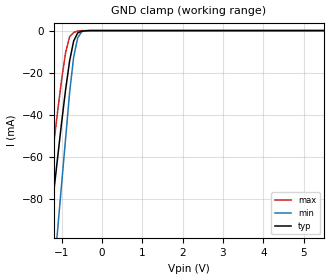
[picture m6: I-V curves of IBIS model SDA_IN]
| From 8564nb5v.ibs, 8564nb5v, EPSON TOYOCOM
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[Model]   SDA_IN
Model_type   Input
Polarity   Non-Inverting
Vinl =   1.5V
Vinh =   3.5V
C_comp   5pF   5pF   5pF
[Temperature Range]   25.00   85.00   -40.00
[Voltage Range]   5.0V   4.5V   5.50V
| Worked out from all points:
|   GND clamp passes 1 mA (typ) near -0.59 V on its own axis
[GND_clamp]
| voltage   I(typ)   I(min)   I(max)
-5.5V     -803.8mA   -1.06A     -733.3mA
-1.5V     -128.2mA   -182.8mA   -102.1mA
-1.4V     -111.3mA   -160.9mA   -86.3mA
-1.3V     -94.4mA    -138.9mA   -70.5mA
-1.1V     -60.7mA    -95.1mA    -38.7mA
-900mV    -28mA      -51.2mA    -10.4mA
-800mV    -14.3mA    -29.2mA    -2.9mA
-700mV    -4.9mA     -12.5mA    -900uA
-600mV    -1.1mA     -3.4mA     -200uA
-500mV    -300uA     -500uA     0A
-400mV    -100uA     -100uA     0A
5.5V      0A         0A         0A
